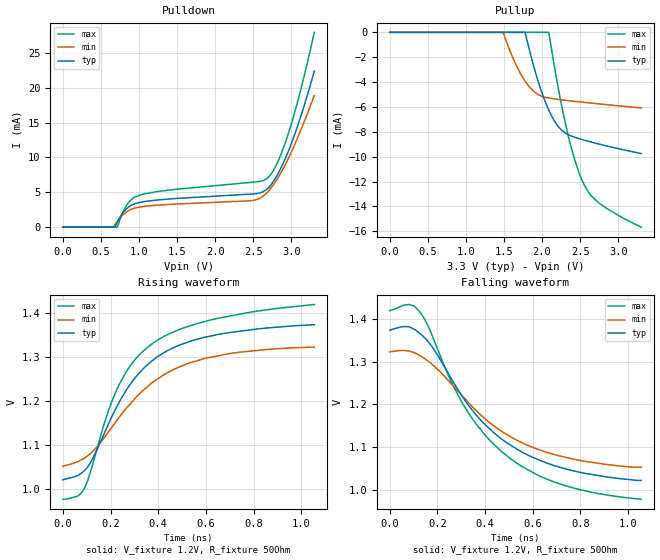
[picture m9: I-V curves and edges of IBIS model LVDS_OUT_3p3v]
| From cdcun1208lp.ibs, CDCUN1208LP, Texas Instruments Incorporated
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[Model]   LVDS_OUT_3p3v
Model_type   Output
Polarity   Non-Inverting
Enable   Active-High
Vmeas = 1.2
Vref = 1.2
Cref = 0pF
Rref = 50
|   typ   min   max
C_comp   5.7061pF   5.6258pF   6.0548pF
[Voltage Range]   3.3   2.97   3.63
[Temperature Range]   27   105   -40
[Pullup Reference]   3.3   2.97   3.63
[Pulldown Reference]   0   0   0
[Power Clamp Reference]   3.3   2.97   3.63
[GND Clamp Reference]   0   0   0
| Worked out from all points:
|   falling waveform, V_fixture 1.2V, R_fixture 50Ohm: 20-80 % time 328ps typ, 344ps min, 324ps max; typ from 1.37 V to 1.02 V
|   rising waveform, V_fixture 1.2V, R_fixture 50Ohm: 20-80 % time 259ps typ, 295ps min, 247ps max; typ from 1.02 V to 1.37 V
[Pulldown]
|   Voltage   I(typ)   I(min)   I(max)
0V        0A         0A         0A
661.7mV   0A         0A         0A
711.3mV   649.1uA    795.4uA    0A
794mV     2.126mA    1.819mA    2.286mA
860.1mV   2.868mA    2.361mA    3.508mA
1.067V    3.658mA    2.975mA    4.763mA
2.448V    4.732mA    3.773mA    6.403mA
2.68V     5.475mA    4.961mA    6.997mA
2.812V    7.432mA    6.887mA    9.157mA
2.953V    10.71mA    9.708mA    13.2mA
3.118V    15.73mA    13.8mA     19.54mA
3.3V      22.39mA    18.88mA    27.95mA
[Pullup]
|   Voltage   I(typ)   I(min)   I(max)
0V        0A         0A         0A
1.489V    0A         -12.88uA   0A
1.613V    0A         -2.006mA   0A
1.77V     0A         -3.865mA   0A
1.944V    -3.853mA   -4.986mA   0A
2.084V    -6.207mA   -5.276mA   0A
2.217V    -7.602mA   -5.395mA   -4.64mA
2.324V    -8.168mA   -5.476mA   -7.824mA
2.432V    -8.444mA   -5.552mA   -10.32mA
2.539V    -8.647mA   -5.624mA   -12.1mA
2.746V    -8.985mA   -5.755mA   -13.72mA
3.3V      -9.748mA   -6.079mA   -15.67mA
[Ramp]
R_load = 50
|   typ   min   max
dV/dt_r   0.211784/2.58604e-010  0.162735/2.94558e-010  0.266114/2.46471e-010
dV/dt_f   0.211784/3.28224e-010  0.162735/3.43634e-010  0.266114/3.23742e-010
[Falling Waveform]
V_fixture = 1.2V
V_fixture_min = 1.2V
V_fixture_max = 1.2V
R_fixture = 50Ohm
C_fixture = 0F
|   Time   V(typ)   V(min)   V(max)
0s        1.374V     1.323V     1.42V
79.64ps   1.382V     1.325V     1.435V
126.2ps   1.367V     1.315V     1.417V
179ps     1.334V     1.293V     1.361V
255.9ps   1.263V     1.25V      1.256V
312.7ps   1.212V     1.215V     1.196V
401.2ps   1.152V     1.166V     1.127V
505.8ps   1.105V     1.124V     1.073V
736.1ps   1.049V     1.076V     1.009V
1.055ns   1.021V     1.052V     976.9mV
[Rising Waveform]
V_fixture = 1.2V
V_fixture_min = 1.2V
V_fixture_max = 1.2V
R_fixture = 50Ohm
C_fixture = 0F
|   Time   V(typ)   V(min)   V(max)
0s        1.021V     1.052V     976.9mV
85.52ps   1.04V      1.069V     997.2mV
121.7ps   1.066V     1.084V     1.05V
185.3ps   1.141V     1.126V     1.169V
226.1ps   1.188V     1.156V     1.226V
294.2ps   1.247V     1.202V     1.289V
365.3ps   1.288V     1.238V     1.327V
461.6ps   1.322V     1.272V     1.357V
593.6ps   1.346V     1.297V     1.381V
1.055ns   1.374V     1.323V     1.42V
